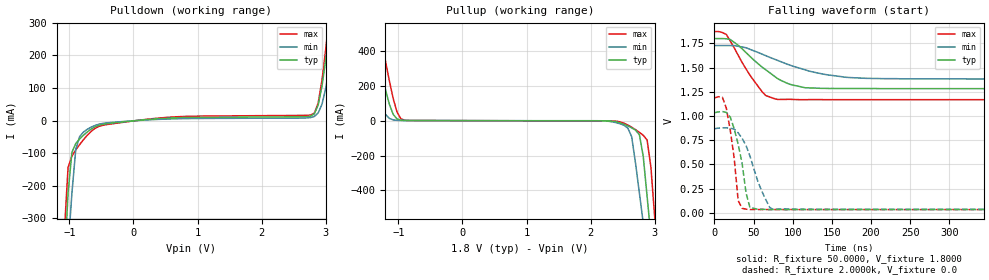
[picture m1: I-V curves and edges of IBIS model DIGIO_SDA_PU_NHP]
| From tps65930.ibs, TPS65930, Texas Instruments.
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|   Model DIGIO_SDA_PU_NHP
[Model]  DIGIO_SDA_PU_NHP
Model_type Output
Polarity   Non-Inverting
Vinl =   0.6300V
Vinh =   1.1700V
C_comp   1.3888pF   2.2766pF   1.3653pF
[Temperature Range]   25.0000   0.1250k   -40.0000
[Pullup Reference]   1.8000V   1.7280V   1.8720V
[Pulldown Reference]   0.0V   0.0V   0.0V
[POWER Clamp Reference]   1.8000V   1.7280V   1.8720V
[GND Clamp Reference]   0.0V   0.0V   0.0V
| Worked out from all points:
|   slope of the pulldown table from 0 to 0.27 V, typ, clamps not added: 56.6 ohm
|   slope of the pullup table from 0 to 0.27 V, typ, clamps not added: 1.35 kohm
|   falling waveform, R_fixture 50.0000, V_fixture 1.8000: 20-80 % time 45.6ns typ, 73.1ns min, 32.2ns max; typ from 1.8 V to 1.28 V
|   falling waveform, R_fixture 2.0000k, V_fixture 0.0: 20-80 % time 13.6ns typ, 21.9ns min, 10.8ns max; typ from 1.03 V to 0.035 V
[Pulldown]
|Voltage   I(typ)   I(min)   I(max)
-1.8V     -3.242A    -2.657A    -3.9A
-1.08V    -451.5mA   -564.9mA   -348.9mA
-1.02V    -222.2mA   -393.4mA   -143.4mA
-960mV    -97.11mA   -222.5mA   -108.3mA
-900mV    -70.41mA   -87.93mA   -89.97mA
-600mV    -19.06mA   -14.77mA   -23.76mA
2.82V     20.66mA    12.68mA    22.74mA
2.94V     105.5mA    50.35mA    124.5mA
3.06V     288.1mA    171.1mA    333.6mA
3.12V     395.6mA    256mA      451.7mA
3.18V     508.5mA    350.3mA    574.2mA
3.6V      68.75A     1.194A     526A
[Pullup]
|Voltage   I(typ)   I(min)   I(max)
-1.8V     68.74A     978.5mA    794.4A
-1.56V    859.4mA    526.7mA    8.216A
-1.44V    613.7mA    323.4mA    854.8mA
-1.32V    384.4mA    148.2mA    583.6mA
-1.14V    94.32mA    12.8mA     228.5mA
-900mV    1.005mA    657.8uA    2.043mA
2.46V     -13.11mA   -18.23mA   -7.345mA
2.64V     -41.51mA   -92.9mA    -37.84mA
2.82V     -205.2mA   -587.1mA   -84.05mA
2.88V     -434mA     -758.8mA   -110.9mA
3V        -893.7mA   -1.103A    -561mA
3.6V      -3.218A    -2.849A    -3.516A
[Ramp]
| variable   typ   min   max
dV/dt_r  0.3744/7.3884n   0.2800/7.7606n   0.4731/6.7469n
dV/dt_f  1.0051/31.3174n   0.9382/51.5796n   1.0598/20.8168n
R_load = 1.0000k
[Falling Waveform]
R_fixture= 50.0000
V_fixture= 1.8000
V_fixture_min= 1.7280
V_fixture_max= 1.8720
|time   V(typ)   V(min)   V(max)
0s        1.8V       1.728V     1.872V
15.15ns   1.798V     1.728V     1.843V
30.3ns    1.731V     1.72V      1.628V
45.45ns   1.615V     1.689V     1.421V
60.61ns   1.507V     1.64V      1.254V
65.66ns   1.477V     1.623V     1.211V
80.81ns   1.386V     1.574V     1.171V
116ns     1.292V     1.477V     1.169V
172ns     1.284V     1.398V     1.169V
500ns     1.283V     1.382V     1.169V
[Falling Waveform]
R_fixture= 2.0000k
V_fixture= 0.0
V_fixture_min= 0.0
V_fixture_max= 0.0
|time   V(typ)   V(min)   V(max)
0s        1.034V     869.1mV    1.187V
15.15ns   1.037V     878.8mV    1.083V
25.25ns   866.8mV    865.7mV    563.1mV
30.3ns    709mV      826.7mV    127.6mV
35.35ns   510.5mV    769.7mV    47.3mV
40.4ns    203.7mV    694.3mV    38.43mV
45.45ns   52.58mV    584.9mV    34.82mV
60.61ns   38.74mV    222.3mV    34.72mV
75.76ns   35.26mV    32.62mV    34.61mV
500ns     34.52mV    37.28mV    34.62mV
